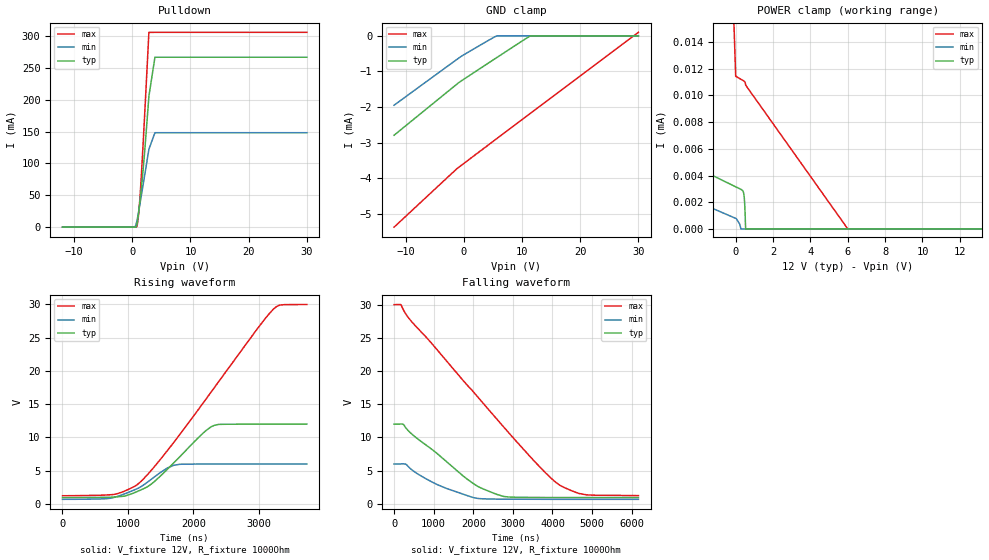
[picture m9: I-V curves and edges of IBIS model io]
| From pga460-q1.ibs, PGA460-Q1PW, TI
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|   io Model
[Model]   io
Model_type   I/O_open_drain
Polarity   Non-Inverting
Vmeas = 6
Vref = 12
Cref = 10pF
Rref = 1000
Vinl=4.8
Vinh=7.2
|   typ   min   max
|   (nom PVT)   (fast PVT)   (slow PVT)
C_comp   2.041e-11   1.831e-11   2.208e-11
| Where nom  PVT is Nominal Process, 12V, 27C
|   Fast PVT is Strong Process,  30V, -40C
|   Slow PVT is Weak Process,   6V, 125C
[Model spec]
|subparameter
|   typ   min   max
Vinl   4.8   2.4   12
Vinh   7.2   3.6   18
[Voltage Range]   12   6   30
|Junction Temperature
[Temperature Range]   27   125   -40
[Pullup Reference]   12   6   30
[Pulldown Reference]   0   0   0
[Power Clamp Reference]   12   6   30
[GND Clamp Reference]   0   0   0
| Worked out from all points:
|   slope of the pulldown table from 0 to 1.8 V, typ, clamps not added: 21.3 ohm
|   falling waveform, V_fixture 12V, R_fixture 1000Ohm: 20-80 % time 1.38us typ, 1.11us min, 2.52us max; typ from 12 V to 0.943 V
|   rising waveform, V_fixture 12V, R_fixture 1000Ohm: 20-80 % time 679ns typ, 519ns min, 1.3us max; typ from 0.942 V to 12 V
[Pulldown]
|   Voltage   I(typ)   I(min)   I(max)
-12V      0A         0A         0A
198mV     0A         0A         0A
516mV     15.92uA    1.371mA    89.43nA
750mV     3.364mA    8.265mA    695.8uA
924mV     11.81mA    15.95mA    7.638mA
1.05V     20.47mA    22.3mA     17.29mA
1.236V    34.79mA    32.2mA     36.77mA
1.44V     51.47mA    43.39mA    64.11mA
2.004V    105.7mA    74.83mA    156mA
2.85V     205.5mA    122.3mA    305.9mA
3.888V    266.9mA    148.3mA    306mA
30V       266.9mA    148.3mA    306mA
[GND Clamp]
|   Voltage   I(typ)   I(min)   I(max)
-12V      -2.793mA   -1.949mA   -5.378mA
-1.17V    -1.353mA   -657.5uA   -3.731mA
5.304V    -646.5uA   -27.33uA   -2.931mA
5.742V    -599.6uA   -55.52nA   -2.877mA
11.41V    -2.47uA    0A         -2.18mA
30V       0A         0A         100.4uA
[POWER Clamp]
|   Voltage   I(typ)   I(min)   I(max)
-12V      11.37uA    8.07uA     1.855A
-3.54V    5.572uA    2.925uA    157.9uA
30mV      3.132uA    766.6nA    11.4uA
204mV     3.013uA    368.9nA    11.27uA
276mV     2.962uA    0A         11.21uA
348mV     2.896uA    0A         11.15uA
420mV     2.678uA    0A         11.09uA
456mV     2.276uA    0A         11.05uA
480mV     1.736uA    0A         11.01uA
528mV     0A         0A         10.77uA
6V        0A         0A         0A
30V       0A         0A         0A
[Ramp]
R_load = 1000
|   typ   min   max
dV/dt_r   6.63303/6.79301e-07   3.18708/5.19063e-07   17.257/1.30018e-06
dV/dt_f   6.63302/1.38273e-06   3.18708/1.11481e-06   17.257/2.51864e-06
[Falling Waveform]
V_fixture = 12V
V_fixture_min = 6V
V_fixture_max = 30V
R_fixture = 1000Ohm
|   Time   V(typ)   V(min)   V(max)
0s        12V        5.999V     29.99V
174.9ns   12.02V     6.018V     29.96V
393ns     10.82V     5.416V     27.8V
1.111us   7.458V     2.852V     23.02V
2.166us   2.478V     792.9mV    15.73V
2.782us   1.107V     711.8mV    11.48V
4.081us   957.5mV    687.6mV    3.262V
4.491us   952.7mV    687.5mV    1.963V
4.859us   949.8mV    687.5mV    1.362V
6.171us   942.9mV    687.4mV    1.247V
[Rising Waveform]
V_fixture = 12V
V_fixture_min = 6V
V_fixture_max = 30V
R_fixture = 1000Ohm
|   Time   V(typ)   V(min)   V(max)
0s        941.8mV    687.4mV    1.227V
800.3ns   1.037V     1.011V     1.452V
1.149us   1.897V     2.328V     2.961V
1.357us   2.993V     3.715V     5.073V
1.701us   6.198V     5.816V     9.283V
2.166us   10.81V     5.987V     15.42V
2.322us   11.83V     5.99V      17.53V
3.229us   11.99V     5.997V     29.37V
3.332us   11.99V     5.997V     29.92V
3.731us   12V        5.997V     29.98V
